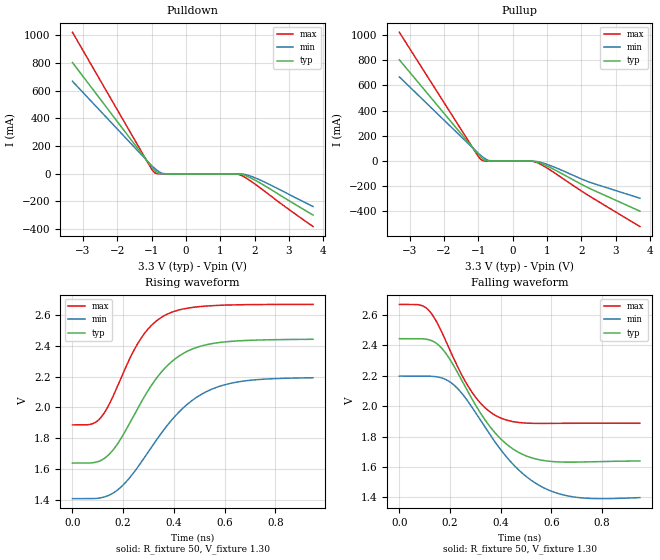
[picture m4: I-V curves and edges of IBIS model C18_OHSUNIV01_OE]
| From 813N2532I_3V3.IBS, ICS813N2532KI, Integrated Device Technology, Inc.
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[Model]   C18_OHSUNIV01_OE
Model_type   Output_ECL
Polarity   Non-Inverting
|   typ   min   max
C_comp   2pF   1.5pF   2.5pF
Vmeas = 2.06V
Rref = 50
Cref = 0
Vref = 1.3V
|   typ   min   max
[Voltage range]   3.3V   3.135V   3.465V
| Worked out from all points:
|   rising waveform, R_fixture 50, V_fixture 1.30: 20-80 % time 189ps typ, 228ps min, 148ps max; typ from 1.64 V to 2.44 V
|   falling waveform, R_fixture 50, V_fixture 1.30: 20-80 % time 182ps typ, 217ps min, 148ps max; typ from 2.44 V to 1.64 V
[Pulldown]
|Voltage   I (typ)   I (min)   I (max)
-3.3V     803.3mA    667.8mA    1.022A
-1V       51.49mA    60.28mA    34.29mA
-891mV    22.12mA    35.72mA    4.841mA
-783mV    3.533mA    15.16mA    219.6uA
-620.9mV  55.04uA    760.2uA    767.7nA
1.323V    -6.972uA   -3.414uA   -32.71uA
1.54V     -1.217mA   -352.5uA   -5.28mA
1.756V    -15.15mA   -7.322mA   -31.31mA
2.134V    -62.65mA   -42.02mA   -96.74mA
3.7V      -298.1mA   -236.4mA   -381.1mA
[Pullup]
|Voltage   I (typ)   I (min)   I (max)
-3.3V     803.3mA    667.8mA    1.022A
-1V       51.49mA    60.28mA    34.29mA
-945mV    35.92mA    47.55mA    16.41mA
-891mV    22.12mA    35.72mA    4.841mA
-783mV    3.533mA    15.16mA    219.6uA
-620.9mV  55.06uA    760.2uA    768.8nA
513.3mV   -454.2uA   -207.8uA   -609.9uA
729.4mV   -10.33mA   -5.625mA   -15.34mA
1.161V    -61.62mA   -43.53mA   -84.29mA
2.242V    -218.4mA   -168.7mA   -280.3mA
3.7V      -398.1mA   -295.5mA   -520.4mA
[Ramp]
|   typ   min   max
dV/dt_r   0.641/0.292n   0.626/0.35n   0.624/0.231n
dV/dt_f   0.648/0.276n   0.644/0.329n   0.625/0.221n
R_load =   50.0000
[Rising Waveform]
R_fixture = 50
V_fixture = 1.30   | VCC_typ - 2V
V_fixture_max = 1.465   | VCC_max - 2V
V_fixture_min = 1.135   | VCC_min - 2V
C_fixture = 0.0p
| Time   typ   min   max
0s        1.64V      1.409V     1.887V
89.39ps   1.644V     1.41V      1.902V
146.4ps   1.699V     1.433V     2.025V
201.6ps   1.827V     1.5V       2.229V
265.3ps   2.017V     1.631V     2.435V
314.8ps   2.151V     1.75V      2.537V
369ps     2.262V     1.873V     2.6V
467.9ps   2.375V     2.04V      2.647V
576.3ps   2.42V      2.135V     2.662V
949ps     2.442V     2.192V     2.668V
[Falling Waveform]
R_fixture = 50
V_fixture = 1.30   | VCC_typ - 2V
V_fixture_max = 1.465   | VCC_max - 2V
V_fixture_min = 1.135   | VCC_min - 2V
C_fixture = 0.0p
| Time   typ   min   max
0s        2.443V     2.197V     2.668V
98.9ps    2.441V     2.197V     2.652V
160.7ps   2.392V     2.188V     2.509V
218.7ps   2.253V     2.134V     2.298V
281.5ps   2.062V     2.005V     2.104V
388ps     1.805V     1.74V      1.931V
494.5ps   1.677V     1.546V     1.889V
606.7ps   1.635V     1.437V     1.887V
733.2ps   1.633V     1.395V     1.888V
949ps     1.64V      1.399V     1.887V
